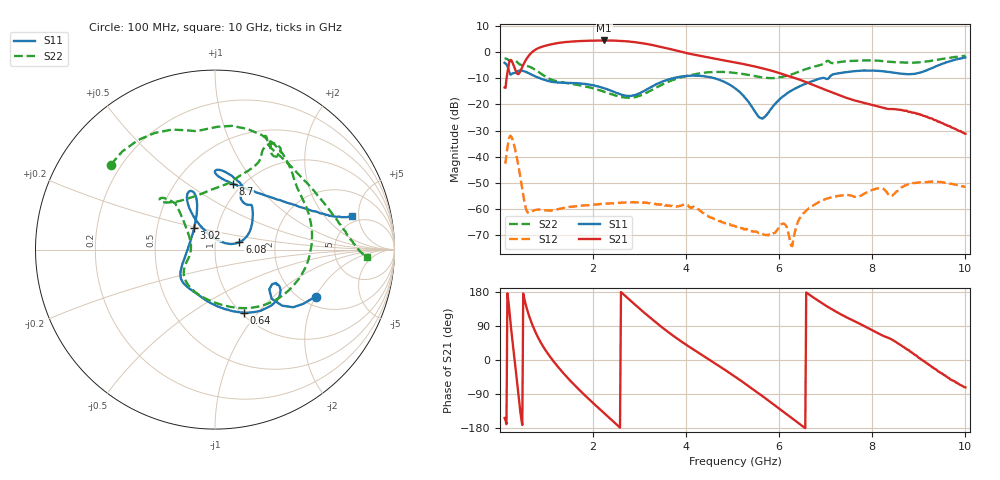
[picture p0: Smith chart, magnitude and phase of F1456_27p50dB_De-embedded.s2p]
! Integrated Device Technology
! Corporate Headquarters
! 6024 Silver Creek Valley Road
! San Jose, CA 95138  USA
! Phone:  1-408-284-8200
! Toll Free:  1-800-223-1366
! Webpage:  http://www.idt.com/
! Timing and RF Division
! 515 Groton Road, Suite 102
! Westford, MA 01886-6024
! Device:  F1456
! Description: 6-bit 0.5 dB Transmit Variable Gain Amplifier
! Frequency:  2100.0 -  2950.00 MHz
! Package:  6x6 mm Thin QFN Plastic Package: 28 pin
! State:  55
! Atten State:  27.5 dB
! Voltage:  +5.00 Volts
! Current:  216.940 mA
! Data:  The device was measured on a the F1455 evaluation board which has
!  individual transmission lines to the RF pins.  Data was collected
!  using a calibrated network analyzer.  The evaluation board was
!  de-embedded using a TRL calibration technique.
!  The reference plane is the edge of the package pin.
!  Pin  1 = CSb
!  Pin  2 = DATA
!  Pin  3 = CLK
!  Pin  4 = RSET
!  Pin  5 = GND
!  Pin  6 = RFIN  = Port 1
!  Pin  7 = GND
!  Pin  8 = NC
!  Pin  9 = NC
!  Pin 10 = NC
!  Pin 11 = NC
!  Pin 12 = NC
!  Pin 13 = NC
!  Pin 14 = /STBY
!  Pin 15 = GND
!  Pin 16 = RFOUT  = Port 2
!  Pin 17 = GND
!  Pin 18 = NC
!  Pin 19 = NC
!  Pin 20 = NC
!  Pin 21 = GND
!  Pin 22 = NC
!  Pin 23 = GND
!  Pin 24 = NC
!  Pin 25 = NC
!  Pin 26 = NC
!  Pin 27 = GND
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# GHz S dB R 50
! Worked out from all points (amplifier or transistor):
!   496 points, 100 MHz to 10 GHz, reference 50 ohm
!   highest |S21| = 4.4 dB at 2.24 GHz (marker M1)
!   |S21| within 3 dB of that: 815.7 MHz to 3.593 GHz (2.777 GHz wide, 126 % of centre)
!   unconditionally stable (mu >= 1): start of sweep to end of sweep
!   at 1.74 GHz: K = 233.76, MAG = 4.7 dB, |S12| = -58.6 dB
!   at 5.06 GHz: K = 1359.92, MAG = -3.1 dB, |S12| = -66.6 dB
!   at 10 GHz: K = 744.02, MAG = -21.5 dB, |S12| = -51.6 dB
!   S11 on the Smith chart (normalised r, x): 100 MHz: 2.37, -2.03; 640 MHz: 1.03, -0.85; 3.02 GHz: 0.77, +0.19; 6.08 GHz: 1.31, +0.11; 8.7 GHz: 0.90, +0.78; 10 GHz: 4.21, +4.12
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0.1  -4.12 -24.9  -13.53 -153.2  -42.30 50.1  -2.52 140.8
0.24  -8.59 -31.2  -3.09 82.3  -32.16 -77.5  -3.45 94.6
0.32  -8.01 -29.0  -6.29 -5.1  -36.64 -155.9  -3.23 67.9
0.42  -7.03 -36.6  -7.92 -119.0  -45.76 139.8  -4.66 40.5
0.52  -7.34 -50.8  -4.21 163.5  -56.65 118.0  -5.06 20.9
0.64  -8.27 -65.5  -0.95 111.4  -61.25 140.9  -5.63 -6.5
0.82  -9.76 -84.0  1.46 59.1  -60.13 119.8  -7.48 -45.1
1.14  -11.43 -110.7  3.09 -1.7  -60.39 84.6  -10.72 -92.5
1.76  -12.03 -139.0  4.22 -85.6  -58.63 49.4  -12.82 -138.8
2.24  -13.82 -154.4  4.42 -140.5  -57.96 31.8  -15.15 -155.9
2.62  -16.34 179.8  4.23 177.2  -57.42 17.6  -17.21 -172.8
3.02  -15.55 134.3  3.47 133.3  -57.54 0.1  -16.53 159.2
3.4  -11.98 113.5  2.21 94.2  -58.03 -15.8  -13.21 139.9
4.1  -9.02 112.6  -0.75 32.4  -59.23 -49.3  -8.81 131.9
5.06  -13.93 122.8  -3.99 -44.8  -66.58 -100.1  -7.96 138.0
5.62  -25.32 66.5  -6.12 -93.5  -69.08 -173.9  -9.63 123.4
6.08  -16.94 16.9  -8.47 -136.0  -65.44 145.8  -9.40 91.0
6.28  -14.53 21.9  -9.59 -154.0  -74.10 158.3  -8.47 78.8
6.7  -11.16 40.8  -12.36 167.8  -58.86 143.2  -5.83 64.9
8.36  -7.63 88.6  -21.76 57.7  -54.70 58.6  -3.72 62.4
8.7  -8.39 74.9  -22.48 31.5  -50.90 66.4  -4.02 51.2
10  -2.09 13.8  -31.16 -72.2  -51.55 -26.9  -1.46 -2.6
